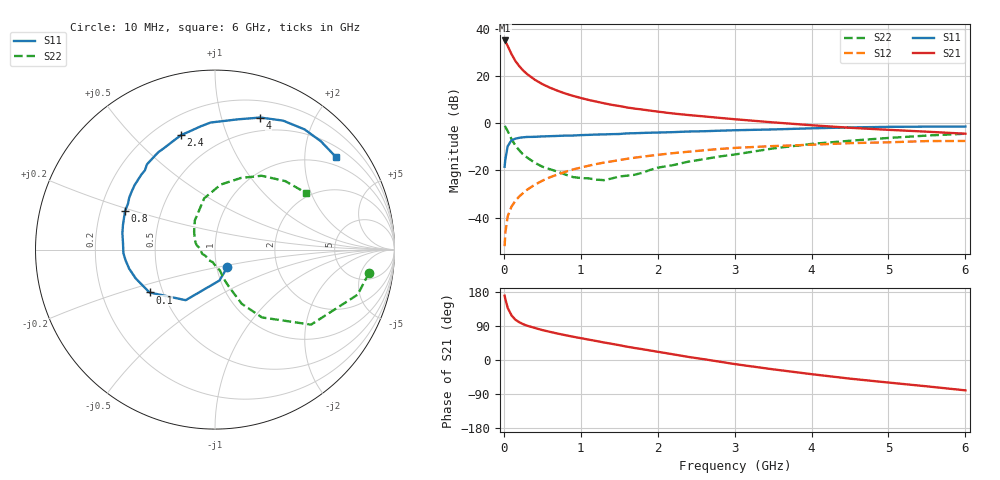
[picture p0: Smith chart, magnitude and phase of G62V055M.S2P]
! SIEMENS Small Signal Semiconductors
! BFG193
! Si NPN RF Bipolar Junction Transistor in SOT223
! VCE = 2 V  IC = 55 mA
! Common Emitter S-Parameters:  August  1996
# GHz  S  MA  R  50
!  f  S11  S21  S12  S22
! GHz  MAG  ANG  MAG  ANG  MAG  ANG  MAG  ANG
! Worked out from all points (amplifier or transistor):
!   36 points, 10 MHz to 6 GHz, reference 50 ohm
!   highest |S21| = 35.0 dB at 10 MHz (marker M1)
!   |S21| within 3 dB of that: start of sweep to 59.82 MHz
!   unconditionally stable (mu >= 1): 333.4 MHz to 2.62 GHz
!   at 250 MHz: K = 0.96, MSG = 25.9 dB, |S12| = -29.6 dB
!   at 1.4 GHz: K = 1.07, MAG = 10.4 dB, |S12| = -16.2 dB
!   at 6 GHz: K = 0.94, MSG = 1.5 dB, |S12| = -7.5 dB
!   S11 on the Smith chart (normalised r, x): 10 MHz: 1.13, -0.22; 100 MHz: 0.42, -0.25; 800 MHz: 0.31, +0.19; 2.4 GHz: 0.31, +0.70; 4 GHz: 0.36, +1.34; 6 GHz: 0.75, +2.76
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0.01  0.12 -54.8  56.17 169.7  0.0025 89.3  0.8678 -8.6
0.02  0.174 -81.8  53.46 160.5  0.0049 78.7  0.8337 -17.5
0.05  0.3258 -120.1  43.02 137.7  0.0107 68.6  0.6792 -38.0
0.1  0.436 -146.8  28.82 117.7  0.0172 65.6  0.4596 -55.3
0.15  0.4698 -159.9  20.67 106.2  0.0228 65.1  0.3369 -63.7
0.2  0.4899 -167.5  16.1 99.7  0.0281 66.3  0.2674 -66.6
0.25  0.5017 -173.1  13.06 94.7  0.0332 67.5  0.2174 -69.6
0.3  0.5108 -177.7  11.01 90.7  0.0388 68.0  0.1891 -71.7
0.4  0.5139 175.9  8.349 84.8  0.0496 68.9  0.146 -74.6
0.5  0.5241 169.9  6.706 79.0  0.0606 67.7  0.1201 -76.8
0.6  0.531 164.9  5.624 74.3  0.0717 66.8  0.1059 -80.7
0.7  0.537 160.7  4.838 69.7  0.0825 65.2  0.0941 -86.6
0.8  0.5456 156.6  4.23 65.5  0.0934 63.1  0.0818 -93.0
1.1  0.5651 145.5  3.104 53.9  0.1255 57.5  0.068 -119.3
1.6  0.6081 128.5  2.15 35.2  0.176 46.3  0.0774 -170.9
2.2  0.6461 111.7  1.602 15.0  0.2321 32.2  0.1293 151.1
2.4  0.6651 106.6  1.486 8.1  0.2489 27.8  0.1535 139.3
3.5  0.7367 80.1  1.039 -24.6  0.3276 0.0  0.292 101.9
4  0.7776 71.1  0.904 -37.4  0.3496 -9.8  0.364 84.9
4.5  0.8125 62.2  0.799 -49.2  0.378 -20.0  0.4244 70.1
5.5  0.8439 45.6  0.66 -69.5  0.4178 -43.1  0.5466 44.3
6  0.8484 37.5  0.598 -80.1  0.42 -56.4  0.5976 31.9
